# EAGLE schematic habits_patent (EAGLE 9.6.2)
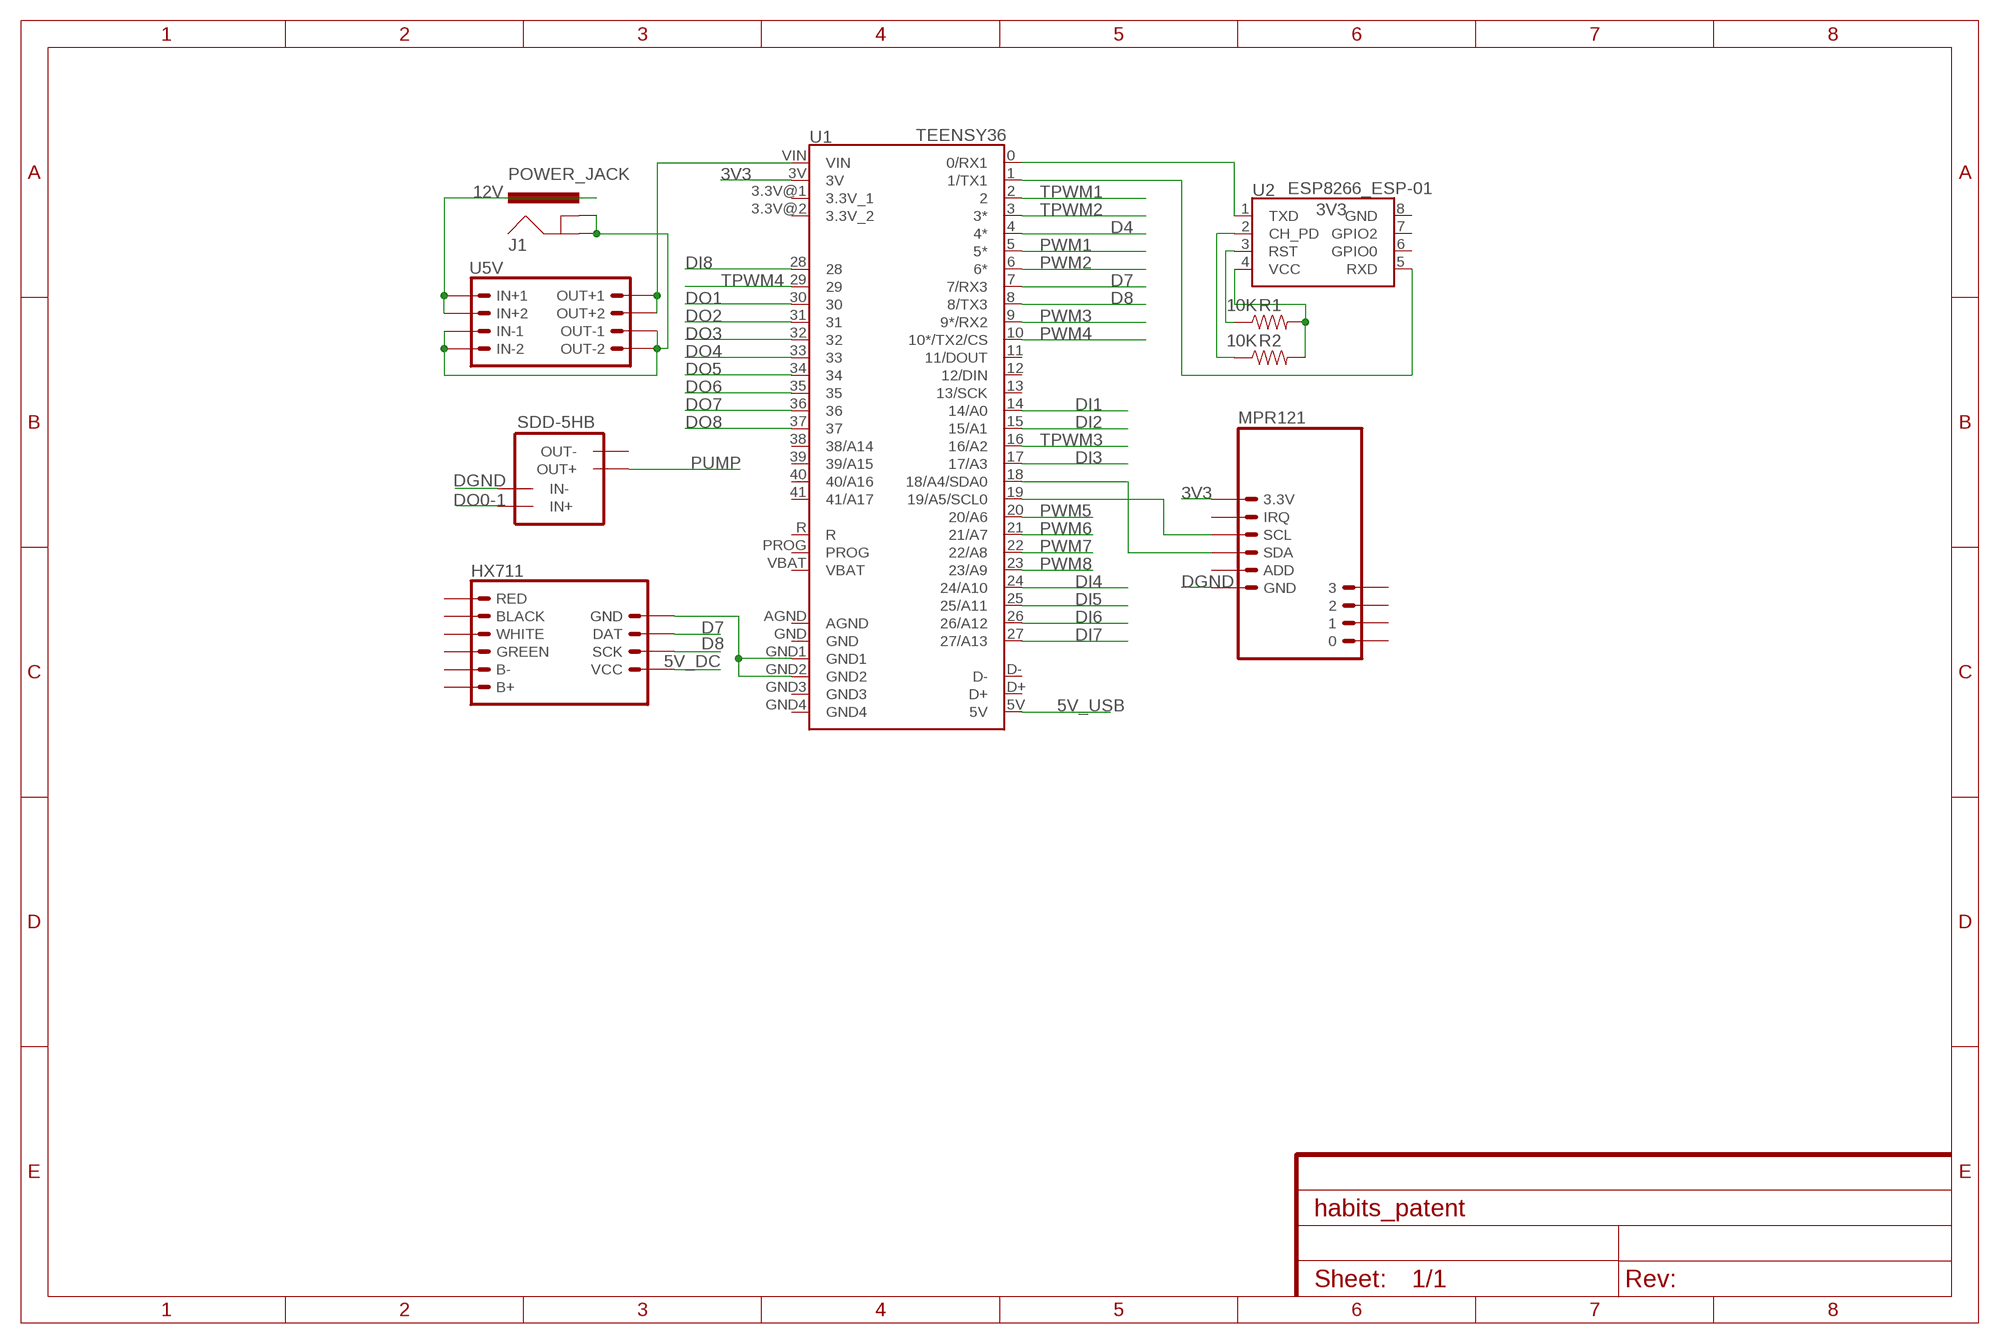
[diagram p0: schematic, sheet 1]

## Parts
J1  POWER_JACK  [POWER_JACK_PTH]
R1  10K  RESISTOR0603  [0603]
R2  10K  RESISTOR0603  [0603]
SDD-5HB  SOLID  [SOLID]
U1  TEENSY36  TEENSY_EXTENDEDW_SILK  [TEENSY_EXTENDED]
U2  ESP8266_ESP-01  [ESP8266_ESP-01]
U3  MPR121_4CH  [MPR121_4CH]
U5V  DC-DC-SMD  [DC-DC-SMD]
U$1  HX711  [HX711]

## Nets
3V3: R1.2 R2.2 U1.3V U2.4(VCC) U3.3.3V
5V_DC: U1.VIN U5V.OUT+1 U5V.OUT+2 U$1.VCC
5V_USB: U1.5V
12V: J1.PWR U5V.IN+1 U5V.IN+2
D4: U1.4(4*)
D7: U1.7(7/RX3) U$1.DAT
D8: U1.8(8/TX3) U$1.SCL(SCK)
DGND: J1.GND J1.GNDBREAK SDD-5HB.2(IN-) U1.GND1 U1.GND2 U3.GND U5V.IN-1 U5V.IN-2 U5V.OUT-1 U5V.OUT-2 U$1.GND
DI1: U1.14(14/A0)
DI2: U1.15(15/A1)
DI3: U1.17(17/A3)
DI4: U1.24(24/A10)
DI5: U1.25(25/A11)
DI6: U1.26(26/A12)
DI7: U1.27(27/A13)
DI8: U1.28
DO0-1: SDD-5HB.1(IN+)
DO1: U1.30
DO2: U1.31
DO3: U1.32
DO4: U1.33
DO5: U1.34
DO6: U1.35
DO7: U1.36
DO8: U1.37
N$1: U1.0(0/RX1) U2.1(TXD)
N$2: U1.1(1/TX1) U2.5(RXD)
N$3: R2.1 U2.2(CH_PD)
N$5: U1.18(18/A4/SDA0) U3.SDA
N$6: R1.1 U2.3(RST)
N$7: U1.19(19/A5/SCL0) U3.SCL
PUMP: SDD-5HB.3(OUT+)
PWM1: U1.5(5*)
PWM2: U1.6(6*)
PWM3: U1.9(9*/RX2)
PWM4: U1.10(10*/TX2/CS)
PWM5: U1.20(20/A6)
PWM6: U1.21(21/A7)
PWM7: U1.22(22/A8)
PWM8: U1.23(23/A9)
TPWM1: U1.2
TPWM2: U1.3(3*)
TPWM3: U1.16(16/A2)
TPWM4: U1.29
Unconnected: SDD-5HB.4(OUT-) U1.11(11/DOUT) U1.12(12/DIN) U1.13(13/SCK) U1.38(38/A14) U1.39(39/A15) U1.40(40/A16) U1.41(41/A17) U1.GND4 U1.PROG U1.R U2.6(GPIO0) U2.7(GPIO2) U2.8(GND) U3.0 U3.1 U3.2 U3.3 U3.ADD U3.IRQ U$1.B+ U$1.B- U$1.BLACK U$1.GREEN U$1.RED U$1.WHITE

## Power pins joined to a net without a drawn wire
3.3V_1: U1.3.3V@1(3.3V_1)
3.3V_2: U1.3.3V@2(3.3V_2)
AGND: U1.AGND
D+: U1.D+
D-: U1.D-
GND: U1.GND
GND3: U1.GND3
VBAT: U1.VBAT

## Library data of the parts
J1 = SparkFun-Connectors:POWER_JACK: Power Jack Connector This is the standard 5.5mm barrel jack for power. The PTH is the most common, proven, reliable, footprint. The Slot footprint only works if the mill layer is transmitted to the PCB fab house so be warned. Here are the connectors we sell at SparkFun: DC Barrel Power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; PROD_ID: CONN-08197
R1 R2 = SparkFun-Resistors:RESISTOR: Generic Resistor Package
SDD-5HB = habits:SOLID
U1 = SparkFun-Boards:TEENSY_EXTENDED: Teensy Footprint Extended Mechanical footprint with connectors for Teensy Development Board with ARM Cortex. SparkFun Products: Teensy 4.1 Teensy 3.6 Teensy 3.5 SparkFun Qwiic Shield for Teensy Extended Teensy Stackable Header Kit (Longer Version)
U2 = SparkFun-RF:ESP8266_ESP-01: ESP8266 ESP-01 Module The ESP8266 WiFi Module is a self contained SOC with integrated TCP/IP protocol stack that can give any microcontroller access to your WiFi network. The ESP8266 is capable of either hosting an application or offloading all Wi-Fi networking functions from another application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; SF_ID: WRL-13678
U3 = habits:MPR121_4CH
U5V = habits:DC-DC-SMD
U$1 = habits:HX711

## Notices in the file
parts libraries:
SparkFun-Boards: Licensing: Creative Commons ShareAlike 4.0 International - https://creativecommons.org/licenses/by-sa/4.0
